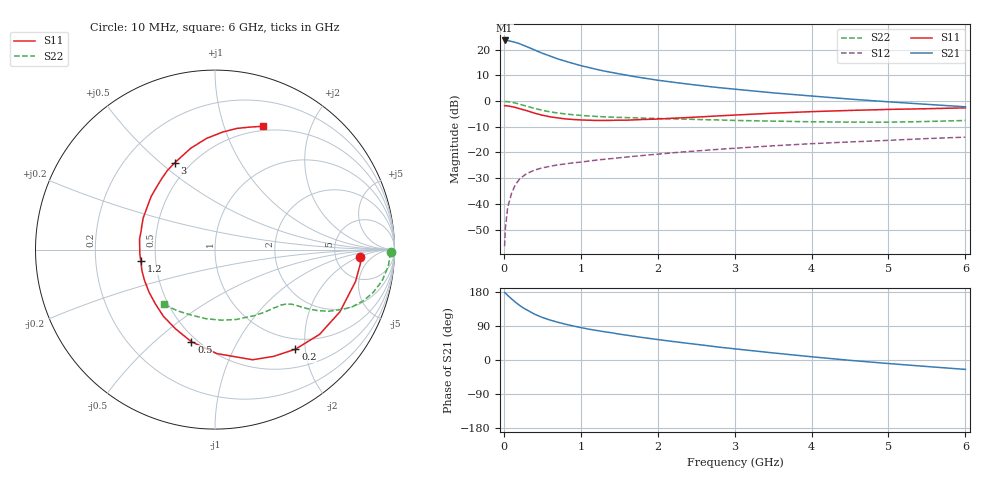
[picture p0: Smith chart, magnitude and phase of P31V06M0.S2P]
! SIEMENS Small Signal Semiconductors
! BFP181
! Si NPN RF Bipolar Junction Transistor in SOT143
! VCE = 1 V  IC = 6 mA
! Common Emitter S-Parameters:  March  1996
# GHz  S  MA  R  50
!  f  S11  S21  S12  S22
! GHz  MAG  ANG  MAG  ANG  MAG  ANG  MAG  ANG
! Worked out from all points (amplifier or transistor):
!   36 points, 10 MHz to 6 GHz, reference 50 ohm
!   highest |S21| = 23.6 dB at 10 MHz (marker M1)
!   |S21| within 3 dB of that: start of sweep to 345.2 MHz
!   unconditionally stable (mu >= 1): 1.156 GHz to end of sweep
!   at 250 MHz: K = 0.29, MSG = 25.5 dB, |S12| = -29.3 dB
!   at 1.4 GHz: K = 1.10, MAG = 14.8 dB, |S12| = -22.4 dB
!   at 6 GHz: K = 1.13, MAG = 3.7 dB, |S12| = -14.1 dB
!   S11 on the Smith chart (normalised r, x): 10 MHz: 8.92, -2.10; 200 MHz: 0.80, -1.81; 500 MHz: 0.47, -0.66; 1.2 GHz: 0.41, -0.07; 3 GHz: 0.41, +0.56; 6 GHz: 0.45, +1.36
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0.01  0.808 -2.9  15.08 178.2  0.0015 88.9  0.9786 -0.9
0.02  0.8141 -5.4  15.07 176.6  0.0034 84.2  0.9755 -2.1
0.05  0.8029 -12.8  15.01 170.5  0.0085 85.1  0.9701 -5.4
0.1  0.7774 -26.5  14.43 161.4  0.016 76.0  0.9471 -10.6
0.15  0.75 -39.0  13.81 152.7  0.0236 70.1  0.9128 -15.2
0.2  0.7132 -51.1  13.11 144.8  0.0297 65.1  0.8737 -19.1
0.25  0.6786 -61.2  12.19 137.7  0.0344 60.4  0.8297 -22.5
0.3  0.6488 -71.1  11.4 132.1  0.0389 56.7  0.7894 -24.9
0.4  0.5797 -88.9  9.854 120.9  0.0454 50.8  0.7181 -28.6
0.5  0.5298 -104.4  8.503 112.3  0.0501 46.6  0.6602 -30.9
0.6  0.4933 -116.5  7.511 105.5  0.0536 44.2  0.6165 -32.4
0.7  0.4698 -127.7  6.605 99.7  0.0573 42.6  0.5847 -33.4
0.9  0.4373 -147.2  5.387 89.9  0.0628 40.8  0.5405 -34.8
1.1  0.4237 -164.0  4.507 81.6  0.0678 40.4  0.5122 -36.4
1.2  0.4184 -171.0  4.145 78.2  0.0708 39.9  0.5019 -37.3
1.7  0.43 161.0  2.984 62.4  0.0843 39.3  0.4703 -42.6
2.2  0.463 140.2  2.323 48.8  0.0984 38.3  0.4493 -49.5
3  0.5329 115.0  1.701 29.5  0.1205 34.5  0.4194 -63.1
3.5  0.5805 103.5  1.443 18.7  0.1345 31.7  0.4065 -73.4
4.5  0.6561 86.3  1.09 -0.9  0.1599 24.8  0.3885 -96.9
5.5  0.7087 74.3  0.862 -17.2  0.1858 18.3  0.3996 -121.2
6  0.7366 68.9  0.772 -24.8  0.1983 14.4  0.4181 -133.1
